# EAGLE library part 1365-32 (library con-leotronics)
DUAL ROW STRAIGHT HEADER 1364 SERIES. 1.27mm x 1.27mm. Without Fixing Post. SMT Source: http://www.leotronics.co.uk/Conexcon/Data%20Sheets/sec.%20A/1364ing.pdf
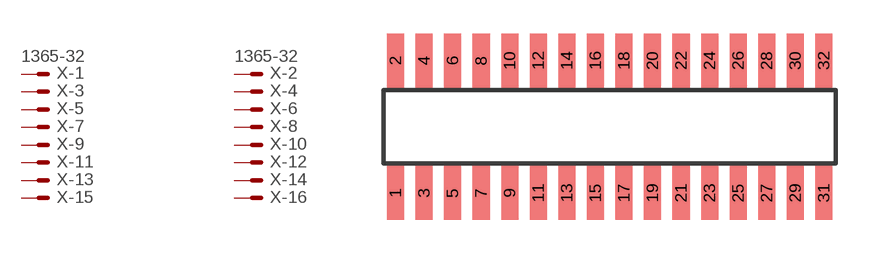
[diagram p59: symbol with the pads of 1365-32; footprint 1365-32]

Designator prefix X; gates -1=MVAL -2=MVAL -3=M -4=M -5=M -6=M -7=M -8=M -9=M -10=M -11=M -12=M -13=M -14=M -15=M -16=M -17=M -18=M -19=M -20=M -21=M -22=M -23=M -24=M -25=M -26=M -27=M -28=M -29=M -30=M -31=M -32=M

## 1365-32 (OC_FARNELL: unknown; OC_NEWARK: unknown)  [1365-32]
1  -1:S  pas
2  -2:S  pas
3  -3:S  pas
4  -4:S  pas
5  -5:S  pas
6  -6:S  pas
7  -7:S  pas
8  -8:S  pas
9  -9:S  pas
10  -10:S  pas
11  -11:S  pas
12  -12:S  pas
13  -13:S  pas
14  -14:S  pas
15  -15:S  pas
16  -16:S  pas
17  -17:S  pas
18  -18:S  pas
19  -19:S  pas
20  -20:S  pas
21  -21:S  pas
22  -22:S  pas
23  -23:S  pas
24  -24:S  pas
25  -25:S  pas
26  -26:S  pas
27  -27:S  pas
28  -28:S  pas
29  -29:S  pas
30  -30:S  pas
31  -31:S  pas
32  -32:S  pas

## Footprint 1365-32 (pad centres in mm)
DUAL ROW STRAIGHT HEADER 1364 SERIES. 1.27mm x 1.27mm. Without Fixing Post. SMT Source: http://www.leotronics.co.uk/Conexcon/Data%20Sheets/sec.%20A/1364ing.pdf
smd 0.76 x 2.4: 1 -9.525,-2.95; 2 -9.525,2.95; 3 -8.255,-2.95; 4 -8.255,2.95; 5 -6.985,-2.95; 6 -6.985,2.95; 7 -5.715,-2.95; 8 -5.715,2.95; 9 -4.445,-2.95; 10 -4.445,2.95; 11 -3.175,-2.95; 12 -3.175,2.95; 13 -1.905,-2.95; 14 -1.905,2.95; 15 -0.635,-2.95; 16 -0.635,2.95; 17 0.635,-2.95; 18 0.635,2.95; 19 1.905,-2.95; 20 1.905,2.95; 21 3.175,-2.95; 22 3.175,2.95; 23 4.445,-2.95; 24 4.445,2.95; 25 5.715,-2.95; 26 5.715,2.95; 27 6.985,-2.95; 28 6.985,2.95; 29 8.255,-2.95; 30 8.255,2.95; 31 9.525,-2.95; 32 9.525,2.95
